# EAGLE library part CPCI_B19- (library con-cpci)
Compact PCI B 19 Source: www.erni.com
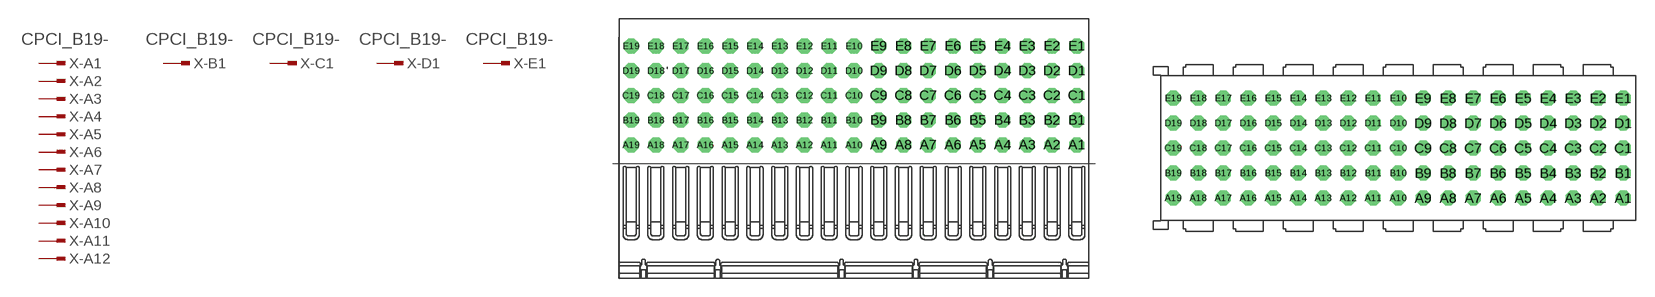
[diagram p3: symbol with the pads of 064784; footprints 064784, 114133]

Designator prefix X; gates -A1=PINV -B1=PINV -C1=PINV -D1=PINV -E1=PINV -A2=PIN -A3=PIN -A4=PIN -A5=PIN -A6=PIN -A7=PIN -A8=PIN -A9=PIN -A10=PIN -A11=PIN -A12=PIN -A13=PIN -A14=PIN -A15=PIN -A16=PIN -A17=PIN -A18=PIN -A19=PIN -B2=PIN -B3=PIN -B4=PIN -B5=PIN -B6=PIN -B7=PIN -B8=PIN -B9=PIN -B10=PIN -B11=PIN -B12=PIN -B13=PIN -B14=PIN -B15=PIN -B16=PIN -B17=PIN -B18=PIN -B19=PIN -C2=PIN -C3=PIN -C4=PIN -C5=PIN -C6=PIN -C7=PIN -C8=PIN -C9=PIN -C10=PIN -C11=PIN -C12=PIN -C13=PIN -C14=PIN -C15=PIN -C16=PIN -C17=PIN -C18=PIN -C19=PIN -D2=PIN -D3=PIN -D4=PIN -D5=PIN -D6=PIN -D7=PIN -D8=PIN -D9=PIN -D10=PIN -D11=PIN -D12=PIN -D13=PIN -D14=PIN -D15=PIN -D16=PIN -D17=PIN -D18=PIN -D19=PIN -E2=PIN -E3=PIN -E4=PIN -E5=PIN -E6=PIN -E7=PIN -E8=PIN -E9=PIN -E10=PIN -E11=PIN -E12=PIN -E13=PIN -E14=PIN -E15=PIN -E16=PIN -E17=PIN -E18=PIN -E19=PIN

## CPCI_B19-064784 (OC_FARNELL: unknown; OC_NEWARK: unknown)  [064784]
A1  -A1:1  in
A2  -A2:1  in
A3  -A3:1  in
A4  -A4:1  in
A5  -A5:1  in
A6  -A6:1  in
A7  -A7:1  in
A8  -A8:1  in
A9  -A9:1  in
A10  -A10:1  in
A11  -A11:1  in
A12  -A12:1  in
A13  -A13:1  in
A14  -A14:1  in
A15  -A15:1  in
A16  -A16:1  in
A17  -A17:1  in
A18  -A18:1  in
A19  -A19:1  in
B1  -B1:1  in
B2  -B2:1  in
B3  -B3:1  in
B4  -B4:1  in
B5  -B5:1  in
B6  -B6:1  in
B7  -B7:1  in
B8  -B8:1  in
B9  -B9:1  in
B10  -B10:1  in
B11  -B11:1  in
B12  -B12:1  in
B13  -B13:1  in
B14  -B14:1  in
B15  -B15:1  in
B16  -B16:1  in
B17  -B17:1  in
B18  -B18:1  in
B19  -B19:1  in
C1  -C1:1  in
C2  -C2:1  in
C3  -C3:1  in
C4  -C4:1  in
C5  -C5:1  in
C6  -C6:1  in
C7  -C7:1  in
C8  -C8:1  in
C9  -C9:1  in
C10  -C10:1  in
C11  -C11:1  in
C12  -C12:1  in
C13  -C13:1  in
C14  -C14:1  in
C15  -C15:1  in
C16  -C16:1  in
C17  -C17:1  in
C18  -C18:1  in
C19  -C19:1  in
D1  -D1:1  in
D2  -D2:1  in
D3  -D3:1  in
D4  -D4:1  in
D5  -D5:1  in
D6  -D6:1  in
D7  -D7:1  in
D8  -D8:1  in
D9  -D9:1  in
D10  -D10:1  in
D11  -D11:1  in
D12  -D12:1  in
D13  -D13:1  in
D14  -D14:1  in
D15  -D15:1  in
D16  -D16:1  in
D17  -D17:1  in
D18  -D18:1  in
D19  -D19:1  in
E1  -E1:1  in
E2  -E2:1  in
E3  -E3:1  in
E4  -E4:1  in
E5  -E5:1  in
E6  -E6:1  in
E7  -E7:1  in
E8  -E8:1  in
E9  -E9:1  in
E10  -E10:1  in
E11  -E11:1  in
E12  -E12:1  in
E13  -E13:1  in
E14  -E14:1  in
E15  -E15:1  in
E16  -E16:1  in
E17  -E17:1  in
E18  -E18:1  in
E19  -E19:1  in

## CPCI_B19-114133 (OC_FARNELL: unknown; OC_NEWARK: unknown)  [114133]
Pads as for 064784

## CPCI_B19-914794 (OC_FARNELL: unknown; OC_NEWARK: unknown)  [914794]
Pads as for 064784

## Footprint 064784 (pad centres in mm)
ERmet Federleiste B 19 / ERmet Female Type B 19 Source: http://www.erni.com/DB/PDF-Drawing/ERmet/064784.pdf
drill 0.7 pad 1.016 octagon: A1 18,0; A2 16,0; A3 14,0; A4 12,0; A5 10,0; A6 8,0; A7 6,0; A8 4,0; A9 2,0; A10 0,0; A11 -2,0; A12 -4,0; A13 -6,0; A14 -8,0; A15 -10,0; A16 -12,0; A17 -14,0; A18 -16,0; A19 -18,0; B1 18,2; B2 16,2; B3 14,2; B4 12,2; B5 10,2; B6 8,2; B7 6,2; B8 4,2; B9 2,2; B10 0,2; B11 -2,2; B12 -4,2; B13 -6,2; B14 -8,2; B15 -10,2; B16 -12,2; B17 -14,2; B18 -16,2; B19 -18,2; C1 18,4; C2 16,4; C3 14,4; C4 12,4; C5 10,4; C6 8,4; C7 6,4; C8 4,4; C9 2,4; C10 0,4; C11 -2,4; C12 -4,4; C13 -6,4; C14 -8,4; C15 -10,4; C16 -12,4; C17 -14,4; C18 -16,4; C19 -18,4; D1 18,6; D2 16,6; D3 14,6; D4 12,6; D5 10,6; D6 8,6; D7 6,6; D8 4,6; D9 2,6; D10 0,6; D11 -2,6; D12 -4,6; D13 -6,6; D14 -8,6; D15 -10,6; D16 -12,6; D17 -14,6; D18 -16,6; D19 -18,6; E1 18,8; E2 16,8; E3 14,8; E4 12,8; E5 10,8; E6 8,8; E7 6,8; E8 4,8; E9 2,8; E10 0,8; E11 -2,8; E12 -4,8; E13 -6,8; E14 -8,8; E15 -10,8; E16 -12,8; E17 -14,8; E18 -16,8; E19 -18,8

## Footprint 114133 (pad centres in mm)
ERmet-FS Federleiste B19 / ERmet-Female Straight Type B19 Source: http://www.erni.com/DB/PDF-Drawing/ERmet/114133.pdf
drill 0.7 pad 1.016 octagon: A1 18,-4; A2 16,-4; A3 14,-4; A4 12,-4; A5 10,-4; A6 8,-4; A7 6,-4; A8 4,-4; A9 2,-4; A10 0,-4; A11 -2,-4; A12 -4,-4; A13 -6,-4; A14 -8,-4; A15 -10,-4; A16 -12,-4; A17 -14,-4; A18 -16,-4; A19 -18,-4; B1 18,-2; B2 16,-2; B3 14,-2; B4 12,-2; B5 10,-2; B6 8,-2; B7 6,-2; B8 4,-2; B9 2,-2; B10 0,-2; B11 -2,-2; B12 -4,-2; B13 -6,-2; B14 -8,-2; B15 -10,-2; B16 -12,-2; B17 -14,-2; B18 -16,-2; B19 -18,-2; C1 18,0; C2 16,0; C3 14,0; C4 12,0; C5 10,0; C6 8,0; C7 6,0; C8 4,0; C9 2,0; C10 0,0; C11 -2,0; C12 -4,0; C13 -6,0; C14 -8,0; C15 -10,0; C16 -12,0; C17 -14,0; C18 -16,0; C19 -18,0; D1 18,2; D2 16,2; D3 14,2; D4 12,2; D5 10,2; D6 8,2; D7 6,2; D8 4,2; D9 2,2; D10 0,2; D11 -2,2; D12 -4,2; D13 -6,2; D14 -8,2; D15 -10,2; D16 -12,2; D17 -14,2; D18 -16,2; D19 -18,2; E1 18,4; E2 16,4; E3 14,4; E4 12,4; E5 10,4; E6 8,4; E7 6,4; E8 4,4; E9 2,4; E10 0,4; E11 -2,4; E12 -4,4; E13 -6,4; E14 -8,4; E15 -10,4; E16 -12,4; E17 -14,4; E18 -16,4; E19 -18,4

## Footprint 914794 (pad centres in mm)
ERmet Federleiste B 19 / ERmet Female Type B 19 Source: http://www.erni.com/DB/PDF-Drawing/ERmet/914794.pdf
drill 0.7 pad 1.016 octagon: A1 18,0; A2 16,0; A3 14,0; A4 12,0; A5 10,0; A6 8,0; A7 6,0; A8 4,0; A9 2,0; A10 0,0; A11 -2,0; A12 -4,0; A13 -6,0; A14 -8,0; A15 -10,0; A16 -12,0; A17 -14,0; A18 -16,0; A19 -18,0; B1 18,2; B2 16,2; B3 14,2; B4 12,2; B5 10,2; B6 8,2; B7 6,2; B8 4,2; B9 2,2; B10 0,2; B11 -2,2; B12 -4,2; B13 -6,2; B14 -8,2; B15 -10,2; B16 -12,2; B17 -14,2; B18 -16,2; B19 -18,2; C1 18,4; C2 16,4; C3 14,4; C4 12,4; C5 10,4; C6 8,4; C7 6,4; C8 4,4; C9 2,4; C10 0,4; C11 -2,4; C12 -4,4; C13 -6,4; C14 -8,4; C15 -10,4; C16 -12,4; C17 -14,4; C18 -16,4; C19 -18,4; D1 18,6; D2 16,6; D3 14,6; D4 12,6; D5 10,6; D6 8,6; D7 6,6; D8 4,6; D9 2,6; D10 0,6; D11 -2,6; D12 -4,6; D13 -6,6; D14 -8,6; D15 -10,6; D16 -12,6; D17 -14,6; D18 -16,6; D19 -18,6; E1 18,8; E2 16,8; E3 14,8; E4 12,8; E5 10,8; E6 8,8; E7 6,8; E8 4,8; E9 2,8; E10 0,8; E11 -2,8; E12 -4,8; E13 -6,8; E14 -8,8; E15 -10,8; E16 -12,8; E17 -14,8; E18 -16,8; E19 -18,8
